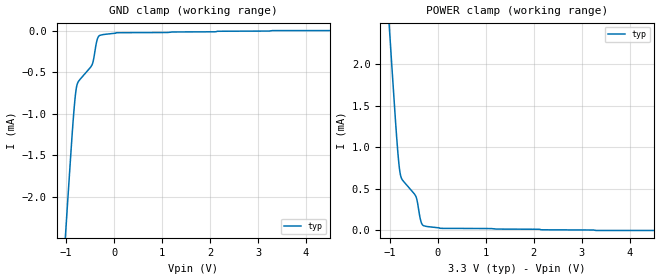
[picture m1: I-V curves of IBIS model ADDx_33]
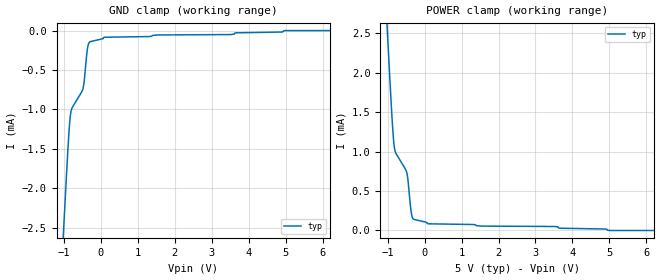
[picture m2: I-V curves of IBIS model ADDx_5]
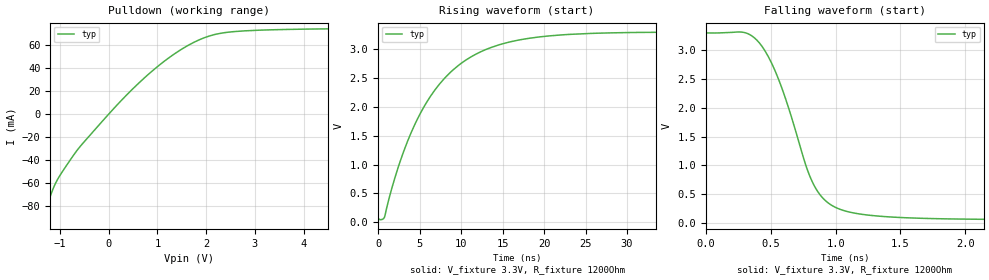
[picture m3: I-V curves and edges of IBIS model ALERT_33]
|Texas Instruments Incorporated
|Digital Temperature Sensor
|   with I2C Interface
| Marketing part#   Digital Voltage Range   Package-type   #pins
|TMP75AID   2.7 to 5.5   SOIC   8
|TMP75AIDG4   2.7 to 5.5   SOIC   8
|TMP75AIDR   2.7 to 5.5   SOIC   8
|TMP75AIDRG4   2.7 to 5.5   SOIC   8
|TMP75AIDGKR   2.7 to 5.5   MSOP   8
|TMP75AIDGKRG4   2.7 to 5.5   MSOP   8
|TMP75AIDGKT   2.7 to 5.5   MSOP   8
|TMP75AIDGKTG4   2.7 to 5.5   MSOP   8
[IBIS Ver]   4.0
[File name]   tmp75.ibs
[File Rev]   1.0
[Date]   12/16/2010
[Source]   Texas Instruments Incorporated.
   Analog-eLab, HPA
   12500 TI Blvd
   Dallas, TX -75243
   For Support e-mail: elab_ibis@list.ti.com
[Notes]   Revision History:
   1.0: 12/16/2010
   - Initial version of the model
   - Model only contains nominal corner (27 degC, nominal
   process) for supply voltages of 3.3V and 5V.
   - Initial Model generated from simulations in TIspiceD
   - Model names with a trailing _33 contains the model for
   3.3V (3V and 3.6V). Model names with trailing _5 contains
   the model for 5V (4.5V and 5.5V) operation.
   - Model not matched to measurements
   - C_comp although listed in numerical order of value are
   obtained from varying PVT conditions. For PVT conditions
   for each specific value refer the buffer description under
   respective [Model]. IBIS model user is responsible for using
   appropriate C_comp to simulate for Signal Integrity.
[Disclaimer]
 This product is designed as an aid for customers of Texas Instruments.
 No warranties, either expressed or implied, with respect to this third
 party software (if any) or with respect to its fitness for any
 particular purpose is claimed by Texas Instruments or the author. The
 software (if any) is provided solely on an "as is" basis. The entire
 risk as to its quality and performance is with the customer
[Copyright] (C) Copyright 2010 Texas Instruments Incorporated.
   All rights reserved.
|   TMP75
[Component]   tmp75d
[Manufacturer] TI
[Package]   |D - SOIC 8-pin
| variable   typ   min   max
R_pkg   0.001403   0.001270   0.001670
L_pkg   1.067772nH 0.952340nH 1.295390nH
C_pkg   0.334850pF 0.307020pF 0.389680pF
[Pin] signal_name  model_name  R_pin  L_pin C_pin
1   SDA   SDA   0.00167  1.29539nH  0.38967pF
2   SCL   SCL   0.00127  0.95242nH  0.30702pF
3   ALERT  ALERT   0.00127  0.95456nH  0.30756pF
4   GND   GND   0.00166  1.29010nH  0.38824pF
5   A2   ADDx   0.00167  1.29535nH  0.38968pF
6   A1   ADDx   0.00127  0.95657nH  0.30813pF
7   A0   ADDx   0.00127  0.95234nH  0.30704pF
8   VP   POWER   0.00167  1.29544nH  0.38965pF
[Component]   tmp75dkr
[Manufacturer] TI
[Package]   |DKR - MSOP 8-pin
| variable   typ   min   max
R_pkg   0.052297   0.048310   0.058660
L_pkg   1.976582nH 1.892000nH 2.124040nH
C_pkg   0.204972pF 0.193670pF 0.210840pF
[Pin] signal_name  model_name  R_pin  L_pin C_pin
1   SDA   SDA   0.05866  2.12404nH  0.19367pF
2   SCL   SCL   0.04975  1.92144nH  0.21084pF
3   ALERT  ALERT   0.04831  1.89200nH  0.21028pF
4   GND   GND   0.05866  2.12418nH  0.19530pF
5   A2   ADDx   0.05866  2.11763nH  0.19387pF
6   A1   ADDx   0.04921  1.90240nH  0.21059pF
7   A0   ADDx   0.04919  1.90198nH  0.21058pF
8   VP   POWER   0.05866  2.11749nH  0.19390pF
|   Model Selectors
[Model Selector]  ADDx
ADDx_33  3.3V digital input
ADDx_5  5V digital input
[Model Selector]  ALERT
ALERT_33  3.3V digital input
ALERT_5  5V digital input
[Model Selector]  SCL
SCL_33   3.3V digital input
SCL_5   5V digital input
[Model Selector]  SDA
SDA_33  3.3V digital I/O open-drain
SDA_5  5V digital I/O open-drain
[Model Selector]  TERM
TERM_33  3.3V anlaog buffers
TERM_5  5V analog buffers
|   TERM 3.3 V Model
[Model] TERM_33
Model_type Terminator
|   typ   min   max
C_comp   1.000e-200   NA   NA
[Voltage Range]   3.3   NA   NA
[Temperature Range]   27   NA   NA
|   TERM 5 V Model
[Model] TERM_5
Model_type Terminator
|   typ   min   max
C_comp   1.000e-200   NA   NA
[Voltage Range]   5   NA   NA
[Temperature Range]   27   NA   NA
| Models and submodels in the file (10): ADDx_33 (Input), ADDx_5 (Input), ALERT_33 (Open_drain), ALERT_5 (Open_drain), SCL_33 (Input), SCL_5 (Input), SDA_33 (I/O_open_drain), SDA_5 (I/O_open_drain), TERM_33 (Terminator), TERM_5 (Terminator)
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|   ADDx 3.3V Model
[Model]   ADDx_33
Model_type   Input
Vinl = 0.66
Vinh = 2.31
|   typ   min   max
C_comp   4.655pF   NA   NA
[Voltage Range]   3.3   NA   NA
[Temperature Range]   27   NA   NA
[Power Clamp Reference]   3.3   NA   NA
[GND Clamp Reference]   -0   NA   NA
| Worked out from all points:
|   GND clamp passes 1 mA (typ) near -0.84 V on its own axis
|   POWER clamp passes 1 mA (typ) near -0.84 V on its own axis
[GND Clamp]
|   Voltage   I(typ)   I(min)   I(max)
-3.3V     -16.09mA   NA         NA
-1.005V   -2.388mA   NA         NA
-866.1mV  -1.181mA   NA         NA
-819.7mV  -847.4uA   NA         NA
-789.3mV  -698.3uA   NA         NA
-740.5mV  -608.9uA   NA         NA
-462.8mV  -415.4uA   NA         NA
-432.6mV  -359.5uA   NA         NA
-354.5mV  -112.5uA   NA         NA
-301.5mV  -58.16uA   NA         NA
65.88mV   -25.49uA   NA         NA
6.59V     0A         NA         NA
[POWER Clamp]
|   Voltage   I(typ)   I(min)   I(max)
-3.3V     16.09mA    NA         NA
-1.005V   2.388mA    NA         NA
-866.1mV  1.181mA    NA         NA
-819.7mV  847.4uA    NA         NA
-789.3mV  698.3uA    NA         NA
-740.5mV  608.9uA    NA         NA
-462.8mV  415.4uA    NA         NA
-432.6mV  359.5uA    NA         NA
-354.5mV  112.5uA    NA         NA
-301.5mV  58.16uA    NA         NA
65.88mV   25.49uA    NA         NA
6.59V     0A         NA         NA
|   ADDx 5V Model
[Model]   ADDx_5
Model_type   Input
Vinl = 1.5
Vinh = 3.5
|   typ   min   max
C_comp   4.58pF   NA   NA
[Voltage Range]   5   NA   NA
[Temperature Range]   27   NA   NA
[Power Clamp Reference]   5   NA   NA
[GND Clamp Reference]   0   NA   NA
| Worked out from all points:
|   GND clamp passes 1 mA (typ) near -0.79 V on its own axis
|   POWER clamp passes 1 mA (typ) near -0.79 V on its own axis
[GND Clamp]
|   Voltage   I(typ)   I(min)   I(max)
-5V       -24.57mA   NA         NA
-1.059V   -2.977mA   NA         NA
-944mV    -1.951mA   NA         NA
-865.2mV  -1.304mA   NA         NA
-813mV    -1.037mA   NA         NA
-481.1mV  -730.8uA   NA         NA
-444.5mV  -611.3uA   NA         NA
-365.9mV  -239.7uA   NA         NA
-292.9mV  -140.9uA   NA         NA
98.01mV   -84.61uA   NA         NA
5.004V    0A         NA         NA
9.985V    0A         NA         NA
[POWER Clamp]
|   Voltage   I(typ)   I(min)   I(max)
-5V       24.57mA    NA         NA
-1.059V   2.977mA    NA         NA
-944mV    1.951mA    NA         NA
-865.2mV  1.304mA    NA         NA
-813mV    1.037mA    NA         NA
-481.1mV  730.8uA    NA         NA
-444.5mV  611.3uA    NA         NA
-365.9mV  239.7uA    NA         NA
-292.9mV  140.9uA    NA         NA
98.01mV   84.61uA    NA         NA
5.004V    0A         NA         NA
9.985V    0A         NA         NA
|   ALERT 3.3V Model
[Model]   ALERT_33
Model_type   Open_drain
Polarity   Non-Inverting
Enable   Active-Low
Vmeas = 1.65
Vref = 1.65
Cref = 15pF
Rref = 1200
|   typ   min   max
C_comp   5.68183e-12  NA   NA
|C_comp (ON state)   1.000e-200   NA   NA
|C_comp (OFF state)   1.000e-200   NA   NA
[Voltage Range]   3.3   NA   NA
[Temperature Range]   27   NA   NA
[Pullup Reference]   3.3   NA   NA
[Pulldown Reference]   0   NA   NA
[Power Clamp Reference]   3.3   NA   NA
[GND Clamp Reference]   0   NA   NA
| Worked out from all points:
|   slope of the pulldown table from 0 to 0.495 V, typ, clamps not added: 22.5 ohm
|   falling waveform, V_fixture 3.3V, R_fixture 1200Ohm: 20-80 % time 291ps typ, NA min, NA max; typ from 3.3 V to 0.058 V
|   rising waveform, V_fixture 3.3V, R_fixture 1200Ohm: 20-80 % time 7.23ns typ, NA min, NA max; typ from 0.058 V to 3.3 V
[Pulldown]
|   Voltage   I(typ)   I(min)   I(max)
-3.3V     -376.2mA   NA         NA
-1.388V   -96.12mA   NA         NA
-1.205V   -72mA      NA         NA
-1.082V   -59.25mA   NA         NA
-731.3mV  -36.24mA   NA         NA
-496.3mV  -23.69mA   NA         NA
263.5mV   12.04mA    NA         NA
852.5mV   35.94mA    NA         NA
1.381V    53.2mA     NA         NA
1.947V    66.06mA    NA         NA
2.797V    72.31mA    NA         NA
6.59V     75.64mA    NA         NA
[Ramp]
R_load = 1200
|   typ   min   max
dV/dt_r   1.94522/7.22568e-009 NA   NA
dV/dt_f   1.94527/2.91171e-010 NA   NA
[Falling Waveform]
V_fixture = 3.3V
R_fixture = 1200Ohm
C_fixture = 0F
|   Time   V(typ)   V(min)   V(max)
0s        3.3V       NA         NA
302.4ps   3.303V     NA         NA
432.2ps   3.065V     NA         NA
507.8ps   2.765V     NA         NA
588.1ps   2.322V     NA         NA
802.3ps   804mV      NA         NA
926.5ps   377.4mV    NA         NA
1.159ns   166.3mV    NA         NA
1.641ns   83.31mV    NA         NA
48.19ns   57.73mV    NA         NA
[Rising Waveform]
V_fixture = 3.3V
R_fixture = 1200Ohm
C_fixture = 0F
|   Time   V(typ)   V(min)   V(max)
0s        57.73mV    NA         NA
762.8ps   88.83mV    NA         NA
1.742ns   637.7mV    NA         NA
3.001ns   1.199V     NA         NA
5.819ns   2.074V     NA         NA
8.69ns    2.597V     NA         NA
12.3ns    2.952V     NA         NA
16.74ns   3.154V     NA         NA
22.05ns   3.248V     NA         NA
48.19ns   3.3V       NA         NA
